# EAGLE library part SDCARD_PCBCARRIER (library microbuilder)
Physical PCB representing an SD Card
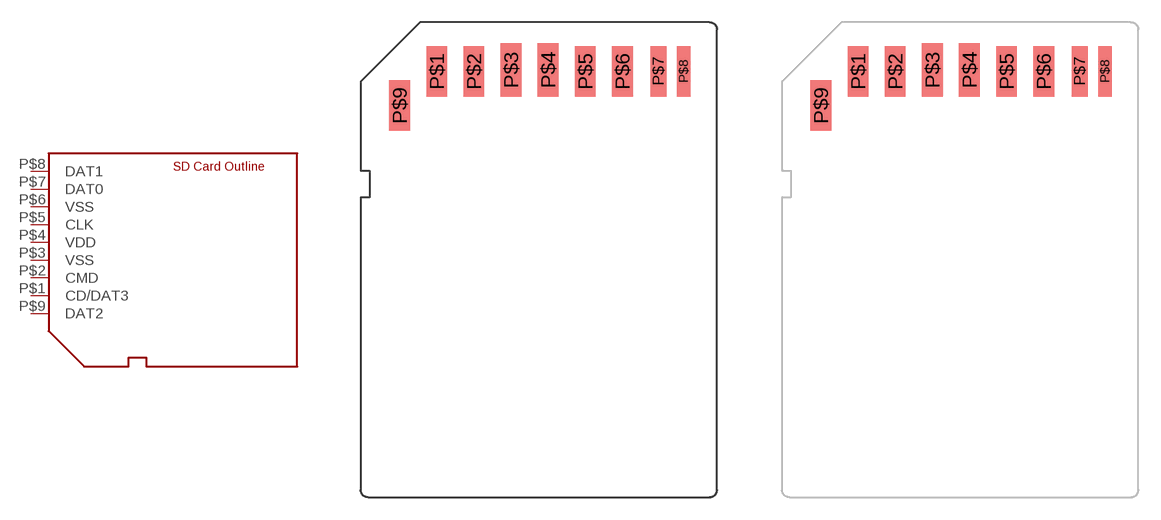
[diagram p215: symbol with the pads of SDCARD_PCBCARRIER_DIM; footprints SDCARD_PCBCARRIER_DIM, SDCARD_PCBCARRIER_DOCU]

Designator prefix -

## SDCARD_PCBCARRIERDIMEN  [SDCARD_PCBCARRIER_DIM]
P$1  CD/DAT3
P$2  CMD
P$3  VSS  pwr
P$4  VDD  pwr
P$5  CLK
P$6  VSS  pwr
P$7  DAT0
P$8  DAT1
P$9  DAT2

## SDCARD_PCBCARRIERTDOCU  [SDCARD_PCBCARRIER_DOCU]
Pads as for SDCARD_PCBCARRIER_DIM

## Footprint SDCARD_PCBCARRIER_DIM (pad centres in mm)
SD Card outline using the dimension layer Source: SD Card Standard v1.9
smd 1.4 x 3.4: P$1 -6.875,0; P$2 -4.375,0; P$5 3.125,0; P$6 5.625,0; P$9 -9.375,-2.3
smd 1.4 x 3.6: P$3 -1.875,0.1; P$4 0.625,0.1
smd 1.1 x 3.4: P$7 8.05,0
smd 0.9 x 3.4: P$8 9.75,0

## Footprint SDCARD_PCBCARRIER_DOCU (pad centres in mm)
smd 1.4 x 3.4: P$1 -6.875,0; P$2 -4.375,0; P$5 3.125,0; P$6 5.625,0; P$9 -9.375,-2.3
smd 1.4 x 3.6: P$3 -1.875,0.1; P$4 0.625,0.1
smd 1.1 x 3.4: P$7 8.05,0
smd 0.9 x 3.4: P$8 9.75,0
